(* Logix 5000 AddOnInstructionDefinition export Banner_Q90R_KD_Param_v4; software revision 33.00; part 2 of 3 *)
(* tags used below, declared in another part *)
   Q90RKD : Banner_Q90RKD_v4;
   Port_Data : Banner_IOL_Port_v4;
   Port : DINT;
   Local_Control : DINT;
   Command_Being_Processed : BOOL;
   Update_Archive : BOOL;
   Index_Write_Inprocess : DINT;
   Index_Write_Control : DINT;
   Inprocess_Index : DINT;
(* Banner_Q90R_KD_Param_v4, continued *)

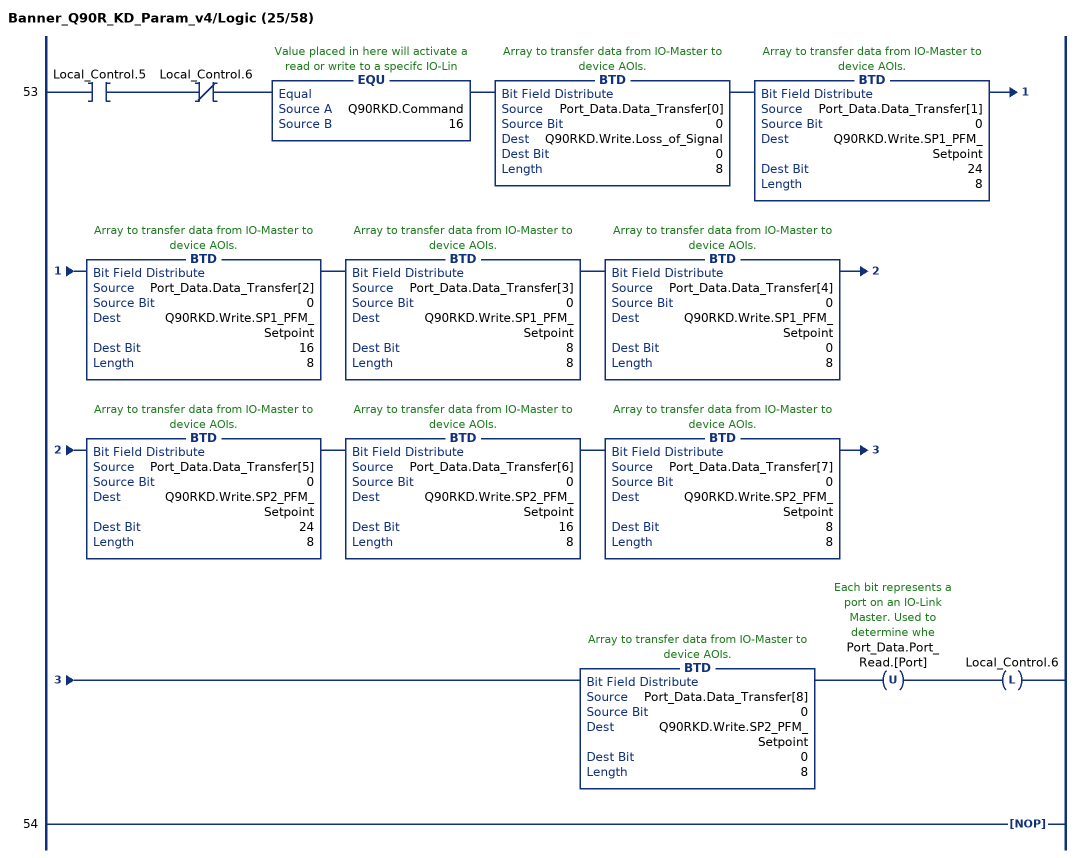
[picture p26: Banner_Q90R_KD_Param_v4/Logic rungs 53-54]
   53: XIC(Local_Control.5)XIO(Local_Control.6)EQU(Q90RKD.Command,16)BTD(Port_Data.Data_Transfer[0],0,Q90RKD.Write.Loss_of_Signal,0,8)BTD(Port_Data.Data_Transfer[1],0,Q90RKD.Write.SP1_PFM_Setpoint,24,8)BTD(Port_Data.Data_Transfer[2],0,Q90RKD.Write.SP1_PFM_Setpoint,16,8)BTD(Port_Data.Data_Transfer[3],0,Q90RKD.Write.SP1_PFM_Setpoint,8,8)BTD(Port_Data.Data_Transfer[4],0,Q90RKD.Write.SP1_PFM_Setpoint,0,8)BTD(Port_Data.Data_Transfer[5],0,Q90RKD.Write.SP2_PFM_Setpoint,24,8)BTD(Port_Data.Data_Transfer[6],0,Q90RKD.Write.SP2_PFM_Setpoint,16,8)BTD(Port_Data.Data_Transfer[7],0,Q90RKD.Write.SP2_PFM_Setpoint,8,8)BTD(Port_Data.Data_Transfer[8],0,Q90RKD.Write.SP2_PFM_Setpoint,0,8)OTU(Port_Data.Port_Read.[Port])OTL(Local_Control.6);
   54: NOP();
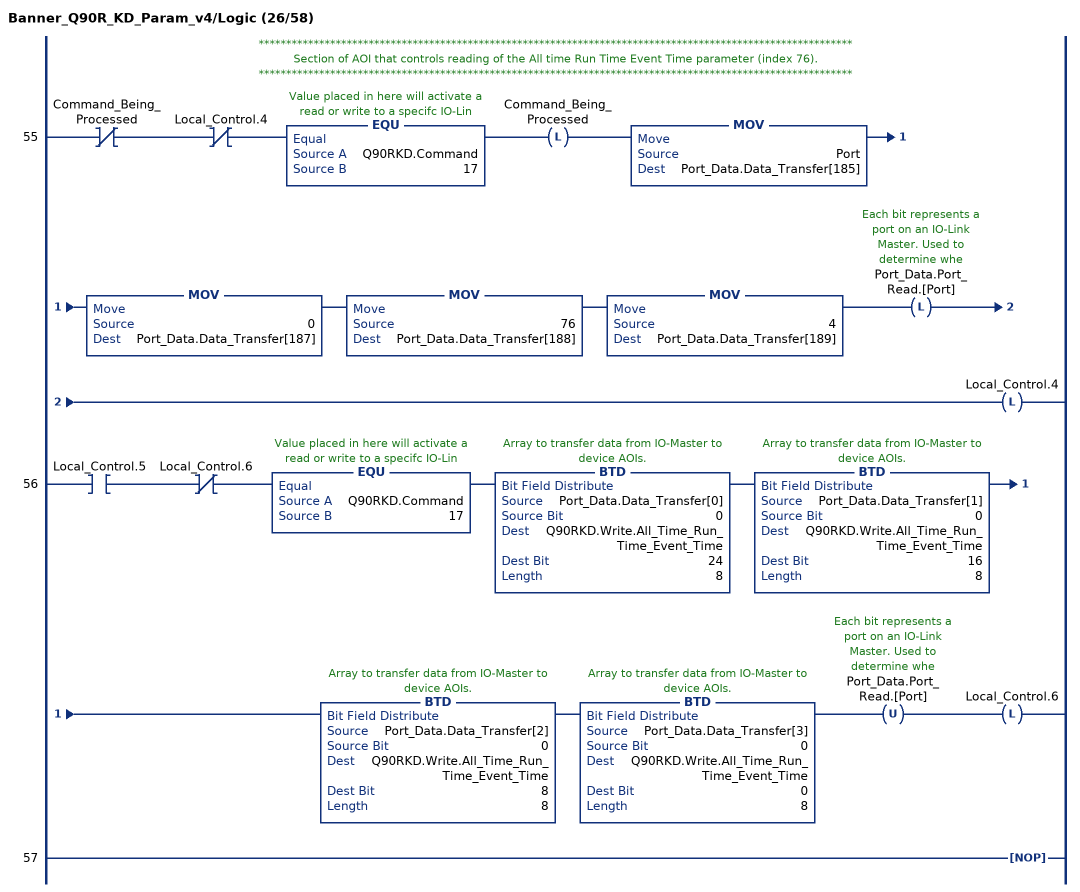
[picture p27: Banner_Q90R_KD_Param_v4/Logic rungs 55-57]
   // ************************************************************************************************************
   // Section of AOI that controls reading of the All time Run Time Event Time parameter (index 76).
   // ************************************************************************************************************
   55: XIO(Command_Being_Processed)XIO(Local_Control.4)EQU(Q90RKD.Command,17)OTL(Command_Being_Processed)MOV(Port,Port_Data.Data_Transfer[185])MOV(0,Port_Data.Data_Transfer[187])MOV(76,Port_Data.Data_Transfer[188])MOV(4,Port_Data.Data_Transfer[189])OTL(Port_Data.Port_Read.[Port])OTL(Local_Control.4);
   56: XIC(Local_Control.5)XIO(Local_Control.6)EQU(Q90RKD.Command,17)BTD(Port_Data.Data_Transfer[0],0,Q90RKD.Write.All_Time_Run_Time_Event_Time,24,8)BTD(Port_Data.Data_Transfer[1],0,Q90RKD.Write.All_Time_Run_Time_Event_Time,16,8)BTD(Port_Data.Data_Transfer[2],0,Q90RKD.Write.All_Time_Run_Time_Event_Time,8,8)BTD(Port_Data.Data_Transfer[3],0,Q90RKD.Write.All_Time_Run_Time_Event_Time,0,8)OTU(Port_Data.Port_Read.[Port])OTL(Local_Control.6);
   57: NOP();
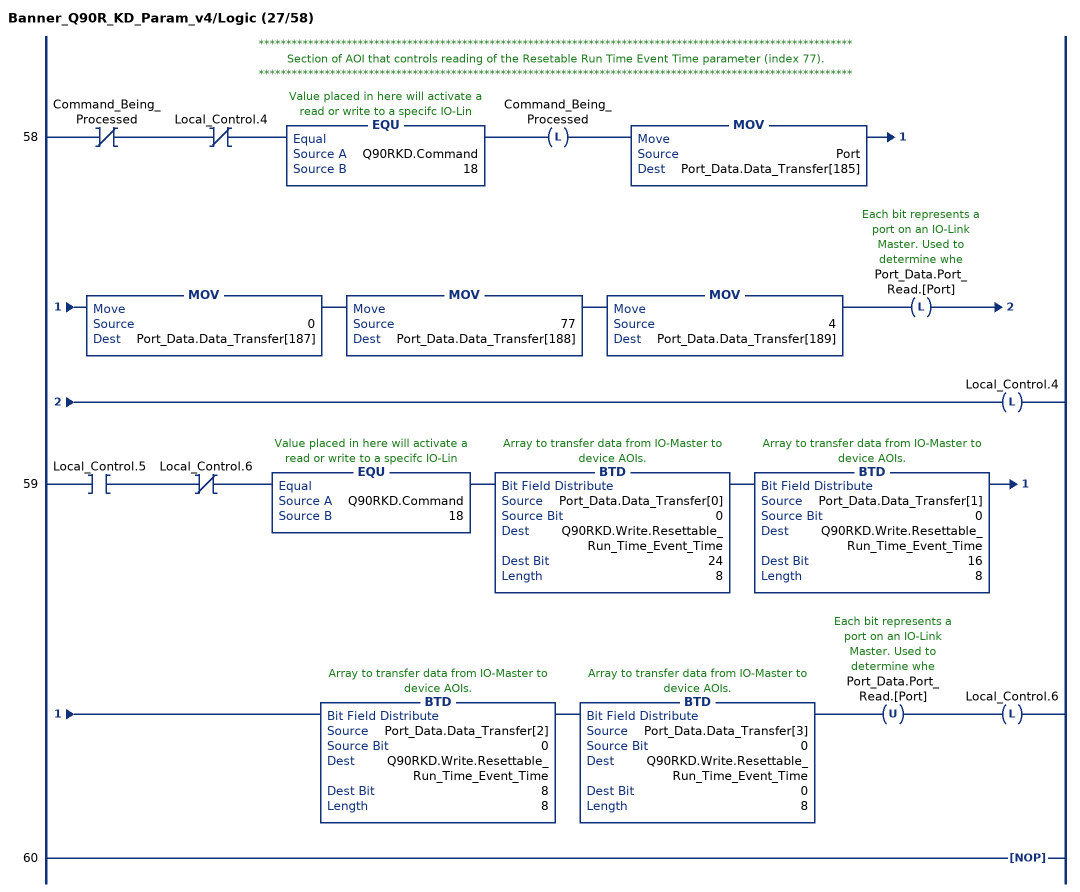
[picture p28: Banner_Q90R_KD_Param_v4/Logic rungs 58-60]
   // ************************************************************************************************************
   // Section of AOI that controls reading of the Resetable Run Time Event Time parameter (index 77).
   // ************************************************************************************************************
   58: XIO(Command_Being_Processed)XIO(Local_Control.4)EQU(Q90RKD.Command,18)OTL(Command_Being_Processed)MOV(Port,Port_Data.Data_Transfer[185])MOV(0,Port_Data.Data_Transfer[187])MOV(77,Port_Data.Data_Transfer[188])MOV(4,Port_Data.Data_Transfer[189])OTL(Port_Data.Port_Read.[Port])OTL(Local_Control.4);
   59: XIC(Local_Control.5)XIO(Local_Control.6)EQU(Q90RKD.Command,18)BTD(Port_Data.Data_Transfer[0],0,Q90RKD.Write.Resettable_Run_Time_Event_Time,24,8)BTD(Port_Data.Data_Transfer[1],0,Q90RKD.Write.Resettable_Run_Time_Event_Time,16,8)BTD(Port_Data.Data_Transfer[2],0,Q90RKD.Write.Resettable_Run_Time_Event_Time,8,8)BTD(Port_Data.Data_Transfer[3],0,Q90RKD.Write.Resettable_Run_Time_Event_Time,0,8)OTU(Port_Data.Port_Read.[Port])OTL(Local_Control.6);
   60: NOP();
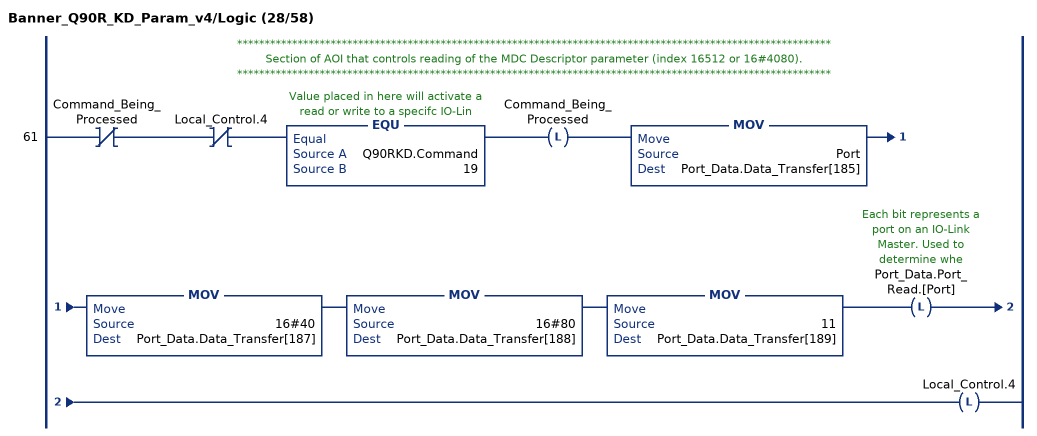
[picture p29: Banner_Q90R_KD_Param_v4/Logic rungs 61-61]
   // ************************************************************************************************************
   // Section of AOI that controls reading of the MDC Descriptor parameter (index 16512 or 16#4080).
   // ************************************************************************************************************
   61: XIO(Command_Being_Processed)XIO(Local_Control.4)EQU(Q90RKD.Command,19)OTL(Command_Being_Processed)MOV(Port,Port_Data.Data_Transfer[185])MOV(16#40,Port_Data.Data_Transfer[187])MOV(16#80,Port_Data.Data_Transfer[188])MOV(11,Port_Data.Data_Transfer[189])OTL(Port_Data.Port_Read.[Port])OTL(Local_Control.4);
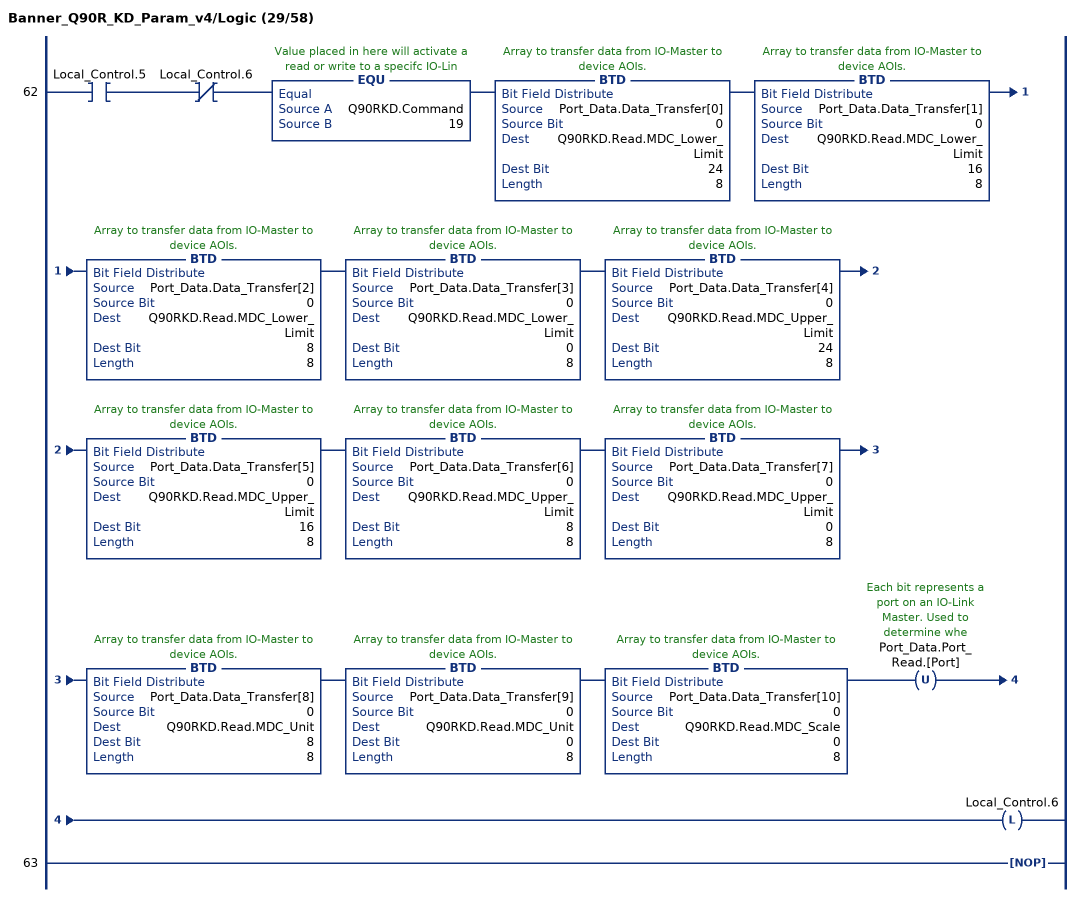
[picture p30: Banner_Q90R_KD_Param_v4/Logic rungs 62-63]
   62: XIC(Local_Control.5)XIO(Local_Control.6)EQU(Q90RKD.Command,19)BTD(Port_Data.Data_Transfer[0],0,Q90RKD.Read.MDC_Lower_Limit,24,8)BTD(Port_Data.Data_Transfer[1],0,Q90RKD.Read.MDC_Lower_Limit,16,8)BTD(Port_Data.Data_Transfer[2],0,Q90RKD.Read.MDC_Lower_Limit,8,8)BTD(Port_Data.Data_Transfer[3],0,Q90RKD.Read.MDC_Lower_Limit,0,8)BTD(Port_Data.Data_Transfer[4],0,Q90RKD.Read.MDC_Upper_Limit,24,8)BTD(Port_Data.Data_Transfer[5],0,Q90RKD.Read.MDC_Upper_Limit,16,8)BTD(Port_Data.Data_Transfer[6],0,Q90RKD.Read.MDC_Upper_Limit,8,8)BTD(Port_Data.Data_Transfer[7],0,Q90RKD.Read.MDC_Upper_Limit,0,8)BTD(Port_Data.Data_Transfer[8],0,Q90RKD.Read.MDC_Unit,8,8)BTD(Port_Data.Data_Transfer[9],0,Q90RKD.Read.MDC_Unit,0,8)BTD(Port_Data.Data_Transfer[10],0,Q90RKD.Read.MDC_Scale,0,8)OTU(Port_Data.Port_Read.[Port])OTL(Local_Control.6);
   63: NOP();
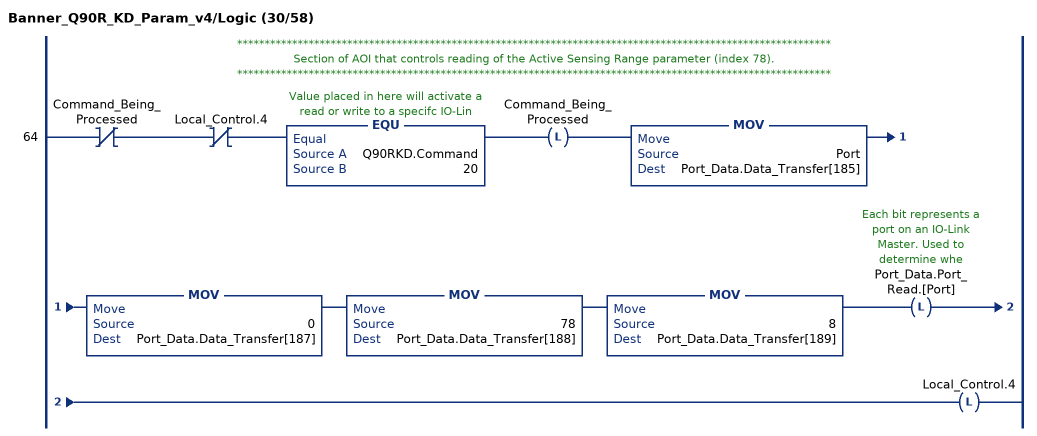
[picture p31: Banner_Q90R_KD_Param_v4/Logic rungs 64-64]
   // ************************************************************************************************************
   // Section of AOI that controls reading of the Active Sensing Range parameter (index 78).
   // ************************************************************************************************************
   64: XIO(Command_Being_Processed)XIO(Local_Control.4)EQU(Q90RKD.Command,20)OTL(Command_Being_Processed)MOV(Port,Port_Data.Data_Transfer[185])MOV(0,Port_Data.Data_Transfer[187])MOV(78,Port_Data.Data_Transfer[188])MOV(8,Port_Data.Data_Transfer[189])OTL(Port_Data.Port_Read.[Port])OTL(Local_Control.4);
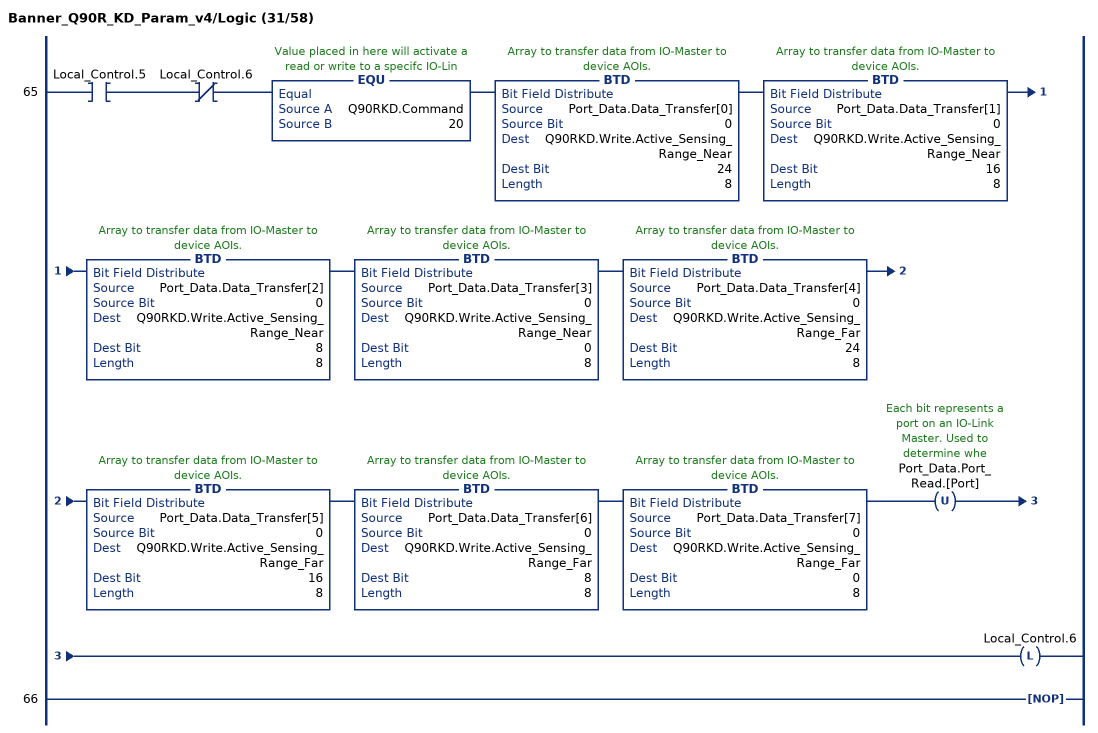
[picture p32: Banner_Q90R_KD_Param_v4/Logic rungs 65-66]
   65: XIC(Local_Control.5)XIO(Local_Control.6)EQU(Q90RKD.Command,20)BTD(Port_Data.Data_Transfer[0],0,Q90RKD.Write.Active_Sensing_Range_Near,24,8)BTD(Port_Data.Data_Transfer[1],0,Q90RKD.Write.Active_Sensing_Range_Near,16,8)BTD(Port_Data.Data_Transfer[2],0,Q90RKD.Write.Active_Sensing_Range_Near,8,8)BTD(Port_Data.Data_Transfer[3],0,Q90RKD.Write.Active_Sensing_Range_Near,0,8)BTD(Port_Data.Data_Transfer[4],0,Q90RKD.Write.Active_Sensing_Range_Far,24,8)BTD(Port_Data.Data_Transfer[5],0,Q90RKD.Write.Active_Sensing_Range_Far,16,8)BTD(Port_Data.Data_Transfer[6],0,Q90RKD.Write.Active_Sensing_Range_Far,8,8)BTD(Port_Data.Data_Transfer[7],0,Q90RKD.Write.Active_Sensing_Range_Far,0,8)OTU(Port_Data.Port_Read.[Port])OTL(Local_Control.6);
   66: NOP();
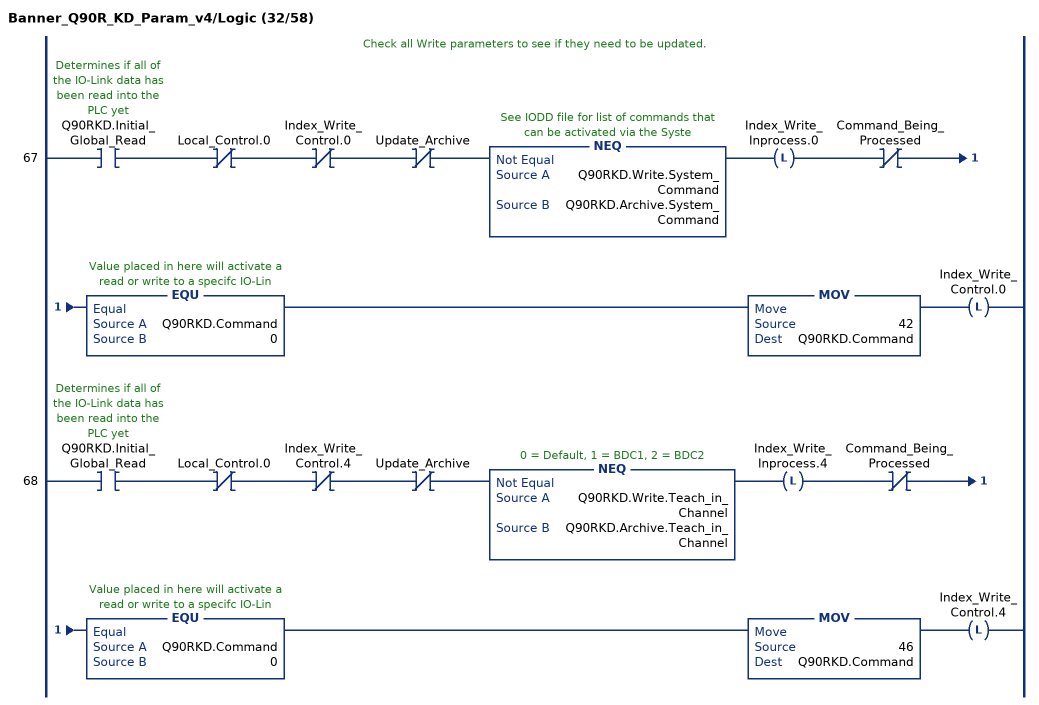
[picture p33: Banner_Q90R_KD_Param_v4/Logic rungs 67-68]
   // Check all Write parameters to see if they need to be updated.
   67: XIC(Q90RKD.Initial_Global_Read)XIO(Local_Control.0)XIO(Index_Write_Control.0)XIO(Update_Archive)NEQ(Q90RKD.Write.System_Command,Q90RKD.Archive.System_Command)OTL(Index_Write_Inprocess.0)XIO(Command_Being_Processed)EQU(Q90RKD.Command,0)MOV(42,Q90RKD.Command)OTL(Index_Write_Control.0);
   68: XIC(Q90RKD.Initial_Global_Read)XIO(Local_Control.0)XIO(Index_Write_Control.4)XIO(Update_Archive)NEQ(Q90RKD.Write.Teach_in_Channel,Q90RKD.Archive.Teach_in_Channel)OTL(Index_Write_Inprocess.4)XIO(Command_Being_Processed)EQU(Q90RKD.Command,0)MOV(46,Q90RKD.Command)OTL(Index_Write_Control.4);
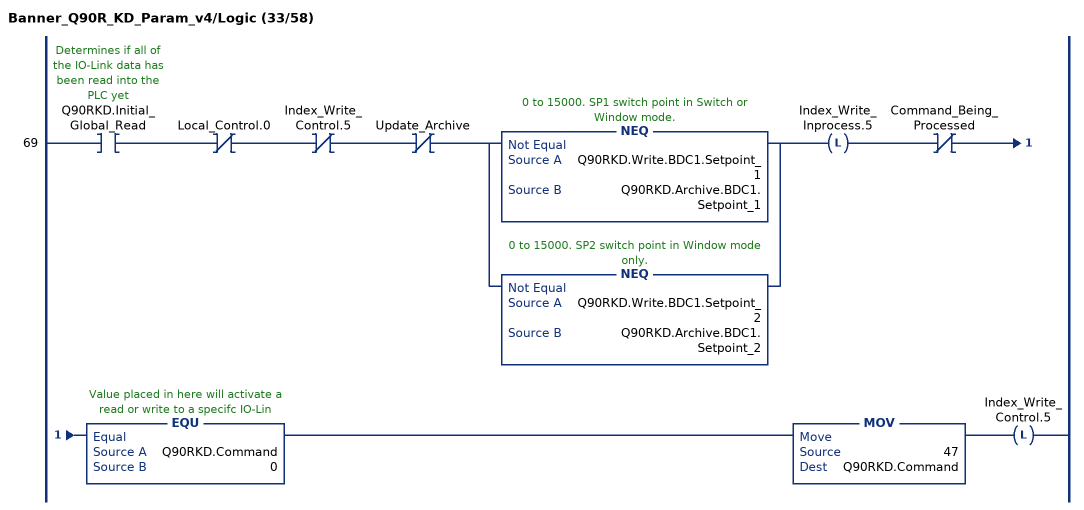
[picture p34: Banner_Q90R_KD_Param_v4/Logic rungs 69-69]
   69: XIC(Q90RKD.Initial_Global_Read)XIO(Local_Control.0)XIO(Index_Write_Control.5)XIO(Update_Archive)[NEQ(Q90RKD.Write.BDC1.Setpoint_1,Q90RKD.Archive.BDC1.Setpoint_1) ,NEQ(Q90RKD.Write.BDC1.Setpoint_2,Q90RKD.Archive.BDC1.Setpoint_2) ]OTL(Index_Write_Inprocess.5)XIO(Command_Being_Processed)EQU(Q90RKD.Command,0)MOV(47,Q90RKD.Command)OTL(Index_Write_Control.5);
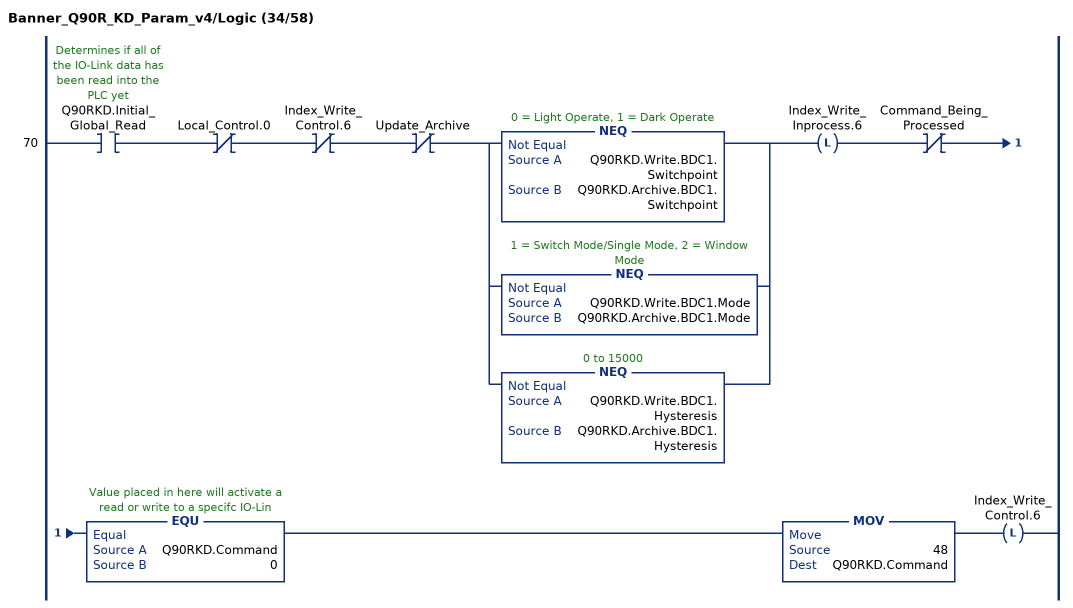
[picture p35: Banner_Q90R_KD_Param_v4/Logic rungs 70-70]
   70: XIC(Q90RKD.Initial_Global_Read)XIO(Local_Control.0)XIO(Index_Write_Control.6)XIO(Update_Archive)[NEQ(Q90RKD.Write.BDC1.Switchpoint,Q90RKD.Archive.BDC1.Switchpoint) ,NEQ(Q90RKD.Write.BDC1.Mode,Q90RKD.Archive.BDC1.Mode) ,NEQ(Q90RKD.Write.BDC1.Hysteresis,Q90RKD.Archive.BDC1.Hysteresis) ]OTL(Index_Write_Inprocess.6)XIO(Command_Being_Processed)EQU(Q90RKD.Command,0)MOV(48,Q90RKD.Command)OTL(Index_Write_Control.6);
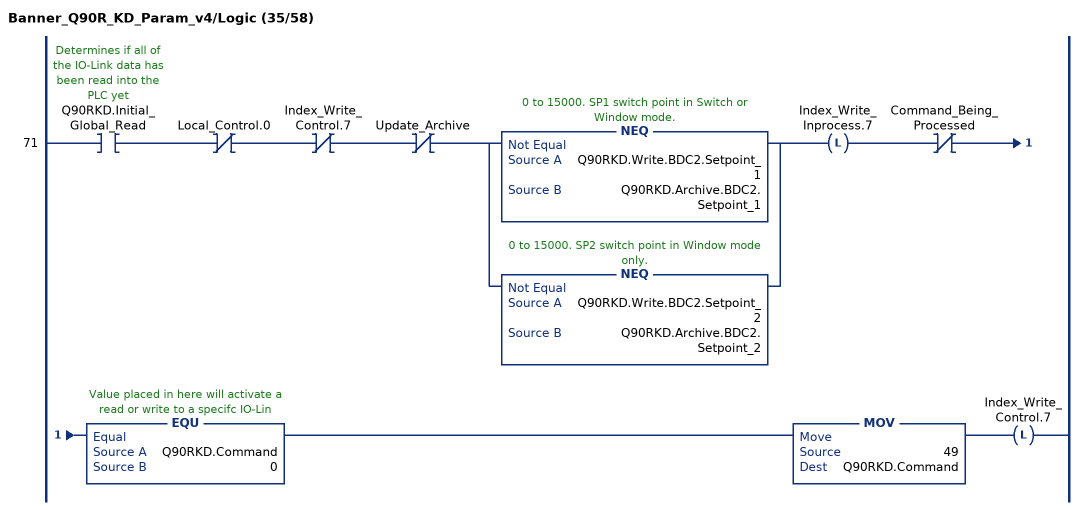
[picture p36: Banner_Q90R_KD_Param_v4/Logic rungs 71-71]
   71: XIC(Q90RKD.Initial_Global_Read)XIO(Local_Control.0)XIO(Index_Write_Control.7)XIO(Update_Archive)[NEQ(Q90RKD.Write.BDC2.Setpoint_1,Q90RKD.Archive.BDC2.Setpoint_1) ,NEQ(Q90RKD.Write.BDC2.Setpoint_2,Q90RKD.Archive.BDC2.Setpoint_2) ]OTL(Index_Write_Inprocess.7)XIO(Command_Being_Processed)EQU(Q90RKD.Command,0)MOV(49,Q90RKD.Command)OTL(Index_Write_Control.7);
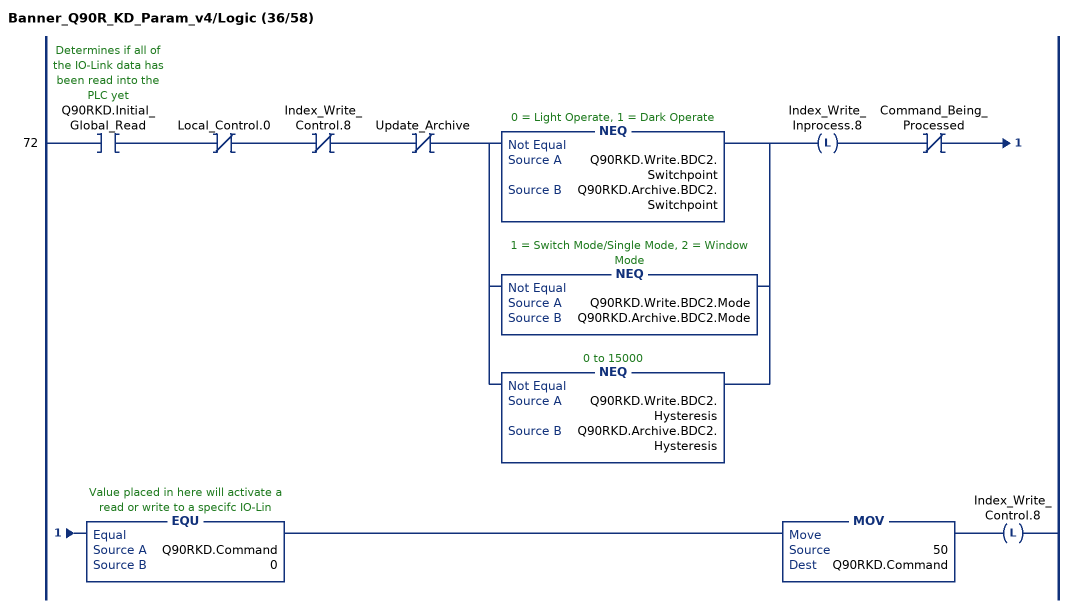
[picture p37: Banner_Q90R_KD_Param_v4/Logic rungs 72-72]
   72: XIC(Q90RKD.Initial_Global_Read)XIO(Local_Control.0)XIO(Index_Write_Control.8)XIO(Update_Archive)[NEQ(Q90RKD.Write.BDC2.Switchpoint,Q90RKD.Archive.BDC2.Switchpoint) ,NEQ(Q90RKD.Write.BDC2.Mode,Q90RKD.Archive.BDC2.Mode) ,NEQ(Q90RKD.Write.BDC2.Hysteresis,Q90RKD.Archive.BDC2.Hysteresis) ]OTL(Index_Write_Inprocess.8)XIO(Command_Being_Processed)EQU(Q90RKD.Command,0)MOV(50,Q90RKD.Command)OTL(Index_Write_Control.8);
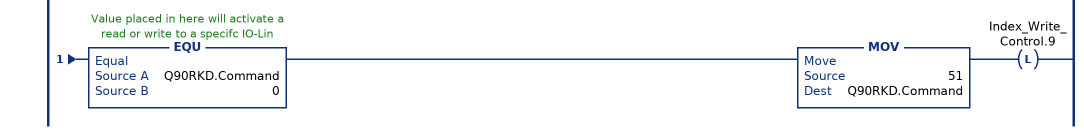
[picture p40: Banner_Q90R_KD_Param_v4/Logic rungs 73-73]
   73: XIC(Q90RKD.Initial_Global_Read)XIO(Local_Control.0)XIO(Index_Write_Control.9)XIO(Update_Archive)[NEQ(Q90RKD.Write.Config.Response_Speed,Q90RKD.Archive.Config.Response_Speed) ,NEQ(Q90RKD.Write.Config.Peak_Select_Mode,Q90RKD.Archive.Config.Peak_Select_Mode) ,NEQ(Q90RKD.Write.Config.Output_Polarity,Q90RKD.Archive.Config.Output_Polarity) ,NEQ(Q90RKD.Write.Config.Process_Data_Filter_Time,Q90RKD.Archive.Config.Process_Data_Filter_Time) ,NEQ(Q90RKD.Write.Config.Process_Data_Layout,Q90RKD.Archive.Config.Process_Data_Layout) ,NEQ(Q90RKD.Write.Config.Remote_Input_Mode,Q90RKD.Archive.Config.Remote_Input_Mode) ,NEQ(Q90RKD.Write.Config.LEDs_Disabled,Q90RKD.Archive.Config.LEDs_Disabled) ,NEQ(Q90RKD.Write.Config.Amplitude_Threshold,Q90RKD.Archive.Config.Amplitude_Threshold) ,NEQ(Q90RKD.Write.Config.Limit_Filter_Enabled,Q90RKD.Archive.Config.Limit_Filter_Enabled) ,NEQ(Q90RKD.Write.Config.Limit_Filter_Positive_Hold_Time,Q90RKD.Archive.Config.Limit_Filter_Positive_Hold_Time) ,NEQ(Q90RKD.Write.Config.Limit_Filter_Negative_Hold_Time,Q90RKD.Archive.Config.Limit_Filter_Negative_Hold_Time) ,NEQ(Q90RKD.Write.Config.Limit_Filter_Positive_Distance,Q90RKD.Archive.Config.Limit_Filter_Positive_Distance) ,NEQ(Q90RKD.Write.Config.Limit_Filter_Negative_Distance,Q90RKD.Archive.Config.Limit_Filter_Negative_Distance) ,NEQ(Q90RKD.Write.Config.Secondary_Output_Mode,Q90RKD.Archive.Config.Secondary_Output_Mode) ]OTL(Index_Write_Inprocess.9)XIO(Command_Being_Processed)EQU(Q90RKD.Command,0)MOV(51,Q90RKD.Command)OTL(Index_Write_Control.9);
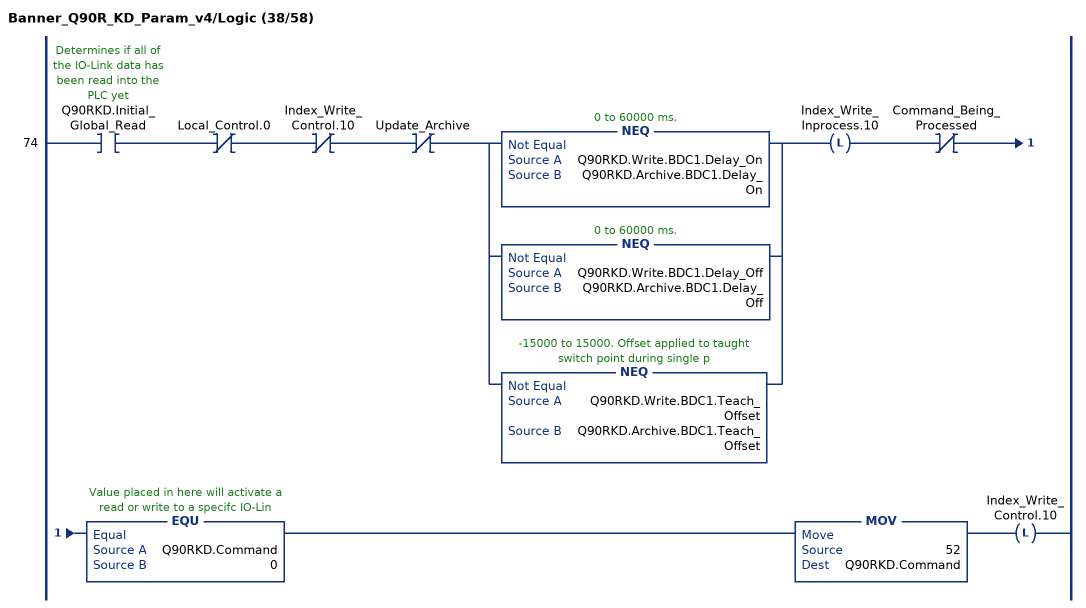
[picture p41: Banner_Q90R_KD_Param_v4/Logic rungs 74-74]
   74: XIC(Q90RKD.Initial_Global_Read)XIO(Local_Control.0)XIO(Index_Write_Control.10)XIO(Update_Archive)[NEQ(Q90RKD.Write.BDC1.Delay_On,Q90RKD.Archive.BDC1.Delay_On) ,NEQ(Q90RKD.Write.BDC1.Delay_Off,Q90RKD.Archive.BDC1.Delay_Off) ,NEQ(Q90RKD.Write.BDC1.Teach_Offset,Q90RKD.Archive.BDC1.Teach_Offset) ]OTL(Index_Write_Inprocess.10)XIO(Command_Being_Processed)EQU(Q90RKD.Command,0)MOV(52,Q90RKD.Command)OTL(Index_Write_Control.10);
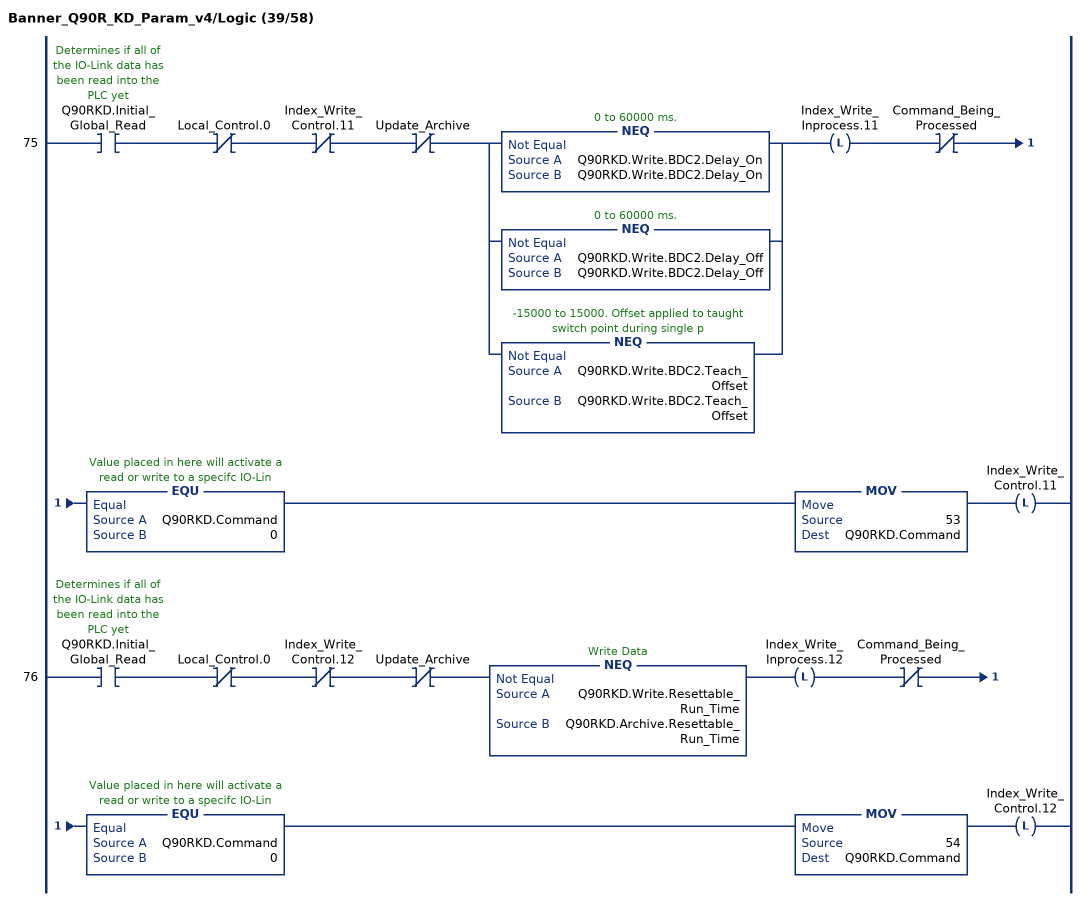
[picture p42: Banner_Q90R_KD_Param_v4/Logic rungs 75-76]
   75: XIC(Q90RKD.Initial_Global_Read)XIO(Local_Control.0)XIO(Index_Write_Control.11)XIO(Update_Archive)[NEQ(Q90RKD.Write.BDC2.Delay_On,Q90RKD.Write.BDC2.Delay_On) ,NEQ(Q90RKD.Write.BDC2.Delay_Off,Q90RKD.Write.BDC2.Delay_Off) ,NEQ(Q90RKD.Write.BDC2.Teach_Offset,Q90RKD.Write.BDC2.Teach_Offset) ]OTL(Index_Write_Inprocess.11)XIO(Command_Being_Processed)EQU(Q90RKD.Command,0)MOV(53,Q90RKD.Command)OTL(Index_Write_Control.11);
   76: XIC(Q90RKD.Initial_Global_Read)XIO(Local_Control.0)XIO(Index_Write_Control.12)XIO(Update_Archive)NEQ(Q90RKD.Write.Resettable_Run_Time,Q90RKD.Archive.Resettable_Run_Time)OTL(Index_Write_Inprocess.12)XIO(Command_Being_Processed)EQU(Q90RKD.Command,0)MOV(54,Q90RKD.Command)OTL(Index_Write_Control.12);
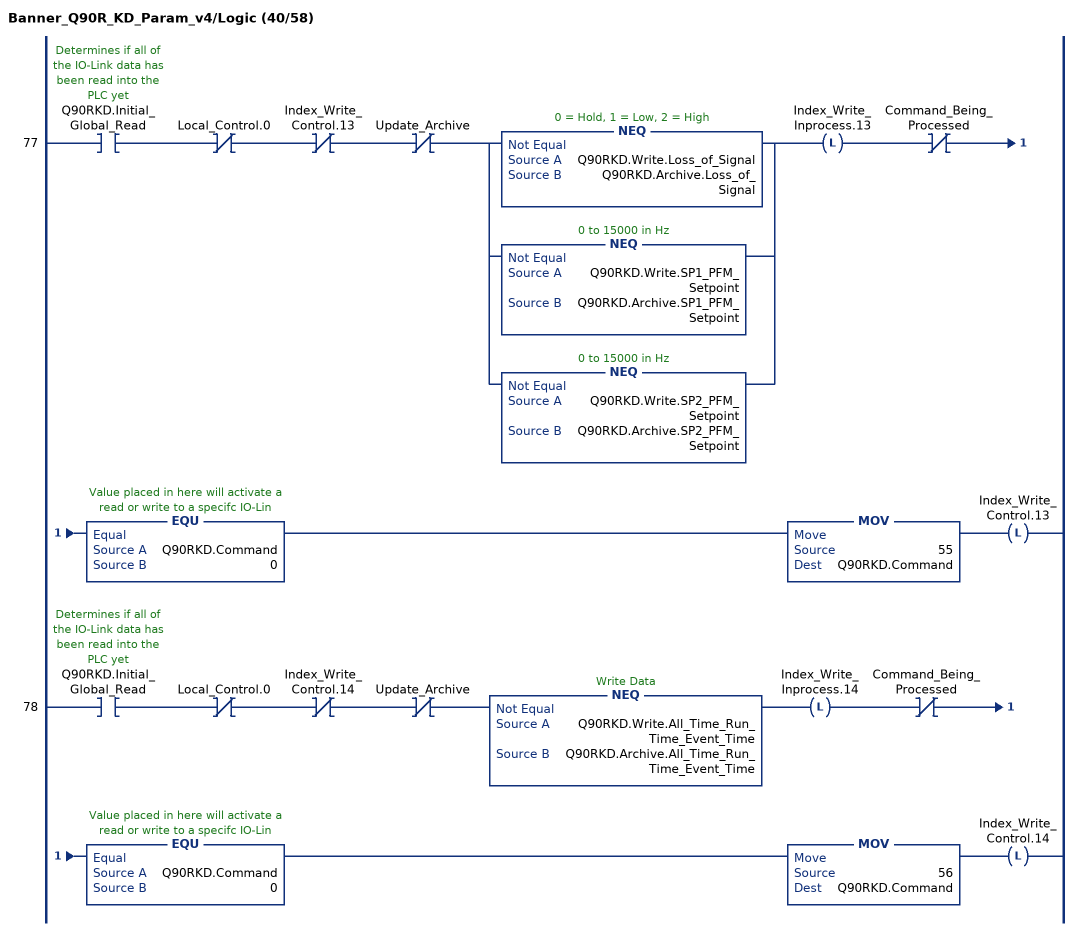
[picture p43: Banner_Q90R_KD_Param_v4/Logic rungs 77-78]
   77: XIC(Q90RKD.Initial_Global_Read)XIO(Local_Control.0)XIO(Index_Write_Control.13)XIO(Update_Archive)[NEQ(Q90RKD.Write.Loss_of_Signal,Q90RKD.Archive.Loss_of_Signal) ,NEQ(Q90RKD.Write.SP1_PFM_Setpoint,Q90RKD.Archive.SP1_PFM_Setpoint) ,NEQ(Q90RKD.Write.SP2_PFM_Setpoint,Q90RKD.Archive.SP2_PFM_Setpoint) ]OTL(Index_Write_Inprocess.13)XIO(Command_Being_Processed)EQU(Q90RKD.Command,0)MOV(55,Q90RKD.Command)OTL(Index_Write_Control.13);
   78: XIC(Q90RKD.Initial_Global_Read)XIO(Local_Control.0)XIO(Index_Write_Control.14)XIO(Update_Archive)NEQ(Q90RKD.Write.All_Time_Run_Time_Event_Time,Q90RKD.Archive.All_Time_Run_Time_Event_Time)OTL(Index_Write_Inprocess.14)XIO(Command_Being_Processed)EQU(Q90RKD.Command,0)MOV(56,Q90RKD.Command)OTL(Index_Write_Control.14);
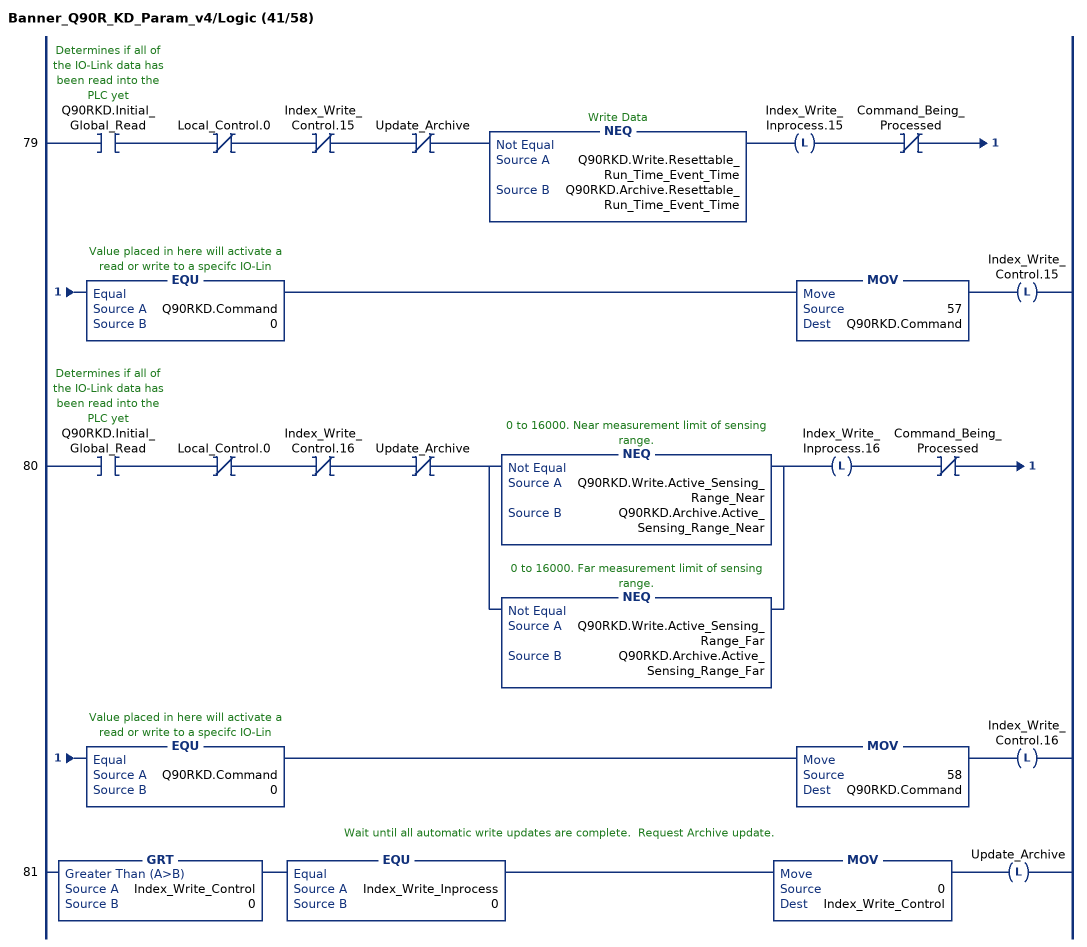
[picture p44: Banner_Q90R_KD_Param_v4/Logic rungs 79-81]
   79: XIC(Q90RKD.Initial_Global_Read)XIO(Local_Control.0)XIO(Index_Write_Control.15)XIO(Update_Archive)NEQ(Q90RKD.Write.Resettable_Run_Time_Event_Time,Q90RKD.Archive.Resettable_Run_Time_Event_Time)OTL(Index_Write_Inprocess.15)XIO(Command_Being_Processed)EQU(Q90RKD.Command,0)MOV(57,Q90RKD.Command)OTL(Index_Write_Control.15);
   80: XIC(Q90RKD.Initial_Global_Read)XIO(Local_Control.0)XIO(Index_Write_Control.16)XIO(Update_Archive)[NEQ(Q90RKD.Write.Active_Sensing_Range_Near,Q90RKD.Archive.Active_Sensing_Range_Near) ,NEQ(Q90RKD.Write.Active_Sensing_Range_Far,Q90RKD.Archive.Active_Sensing_Range_Far) ]OTL(Index_Write_Inprocess.16)XIO(Command_Being_Processed)EQU(Q90RKD.Command,0)MOV(58,Q90RKD.Command)OTL(Index_Write_Control.16);
   // Wait until all automatic write updates are complete.  Request Archive update.
   81: GRT(Index_Write_Control,0)EQU(Index_Write_Inprocess,0)MOV(0,Index_Write_Control)OTL(Update_Archive);
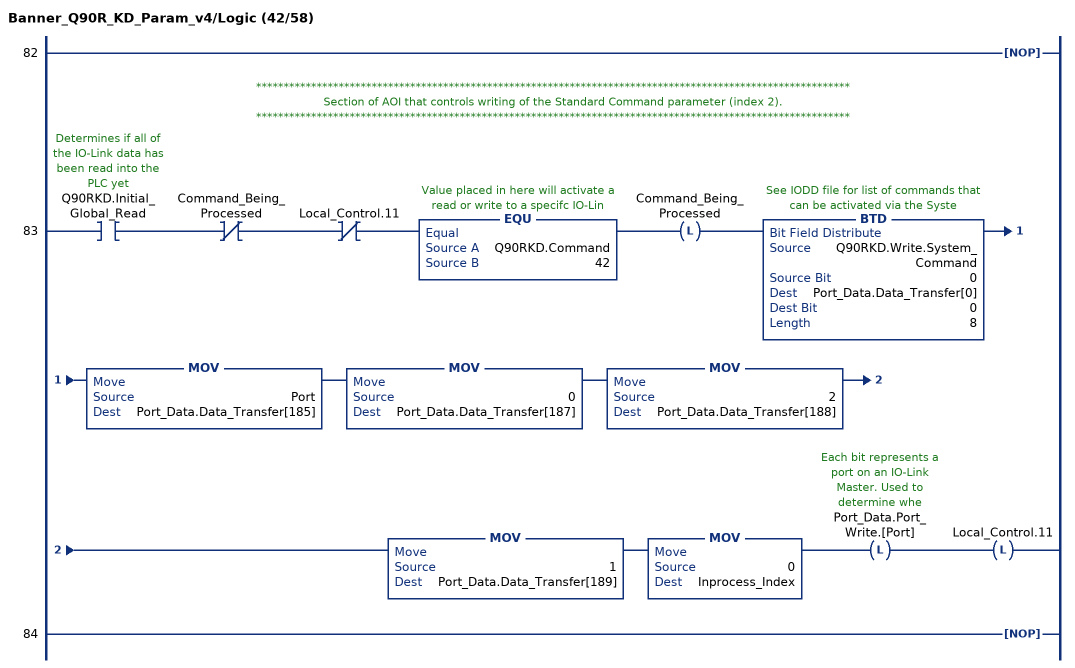
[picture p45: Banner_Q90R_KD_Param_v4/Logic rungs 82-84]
   82: NOP();
   // ************************************************************************************************************
   // Section of AOI that controls writing of the Standard Command parameter (index 2).
   // ************************************************************************************************************
   83: XIC(Q90RKD.Initial_Global_Read)XIO(Command_Being_Processed)XIO(Local_Control.11)EQU(Q90RKD.Command,42)OTL(Command_Being_Processed)BTD(Q90RKD.Write.System_Command,0,Port_Data.Data_Transfer[0],0,8)MOV(Port,Port_Data.Data_Transfer[185])MOV(0,Port_Data.Data_Transfer[187])MOV(2,Port_Data.Data_Transfer[188])MOV(1,Port_Data.Data_Transfer[189])MOV(0,Inprocess_Index)OTL(Port_Data.Port_Write.[Port])OTL(Local_Control.11);
   84: NOP();
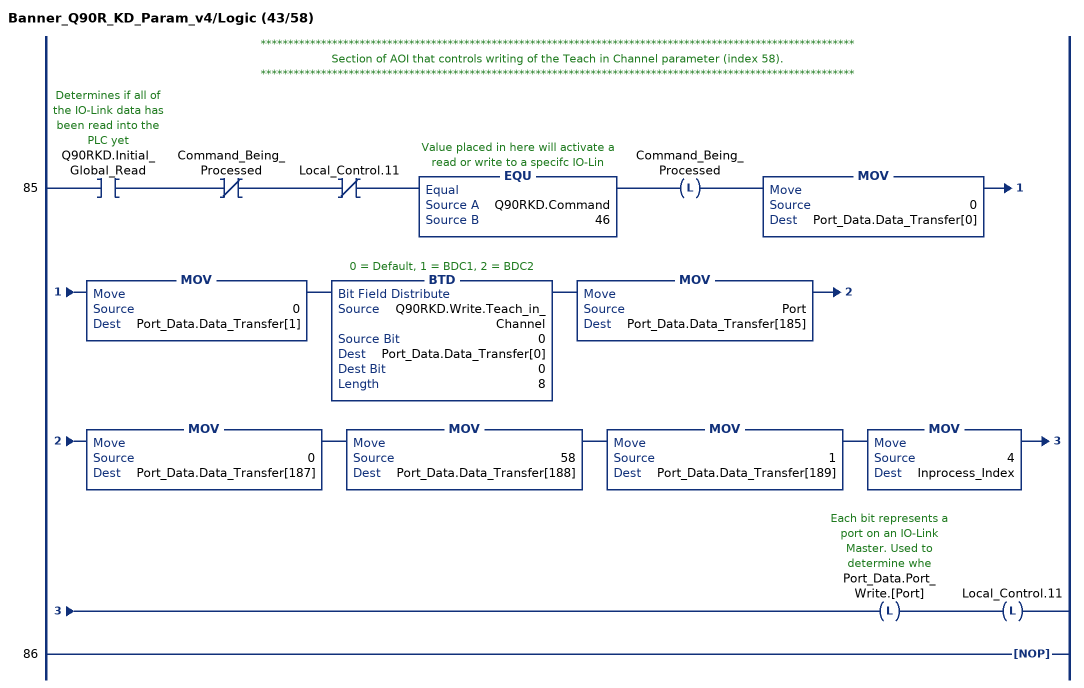
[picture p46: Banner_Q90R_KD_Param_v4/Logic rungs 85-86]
   // ************************************************************************************************************
   // Section of AOI that controls writing of the Teach in Channel parameter (index 58).
   // ************************************************************************************************************
   85: XIC(Q90RKD.Initial_Global_Read)XIO(Command_Being_Processed)XIO(Local_Control.11)EQU(Q90RKD.Command,46)OTL(Command_Being_Processed)MOV(0,Port_Data.Data_Transfer[0])MOV(0,Port_Data.Data_Transfer[1])BTD(Q90RKD.Write.Teach_in_Channel,0,Port_Data.Data_Transfer[0],0,8)MOV(Port,Port_Data.Data_Transfer[185])MOV(0,Port_Data.Data_Transfer[187])MOV(58,Port_Data.Data_Transfer[188])MOV(1,Port_Data.Data_Transfer[189])MOV(4,Inprocess_Index)OTL(Port_Data.Port_Write.[Port])OTL(Local_Control.11);
   86: NOP();
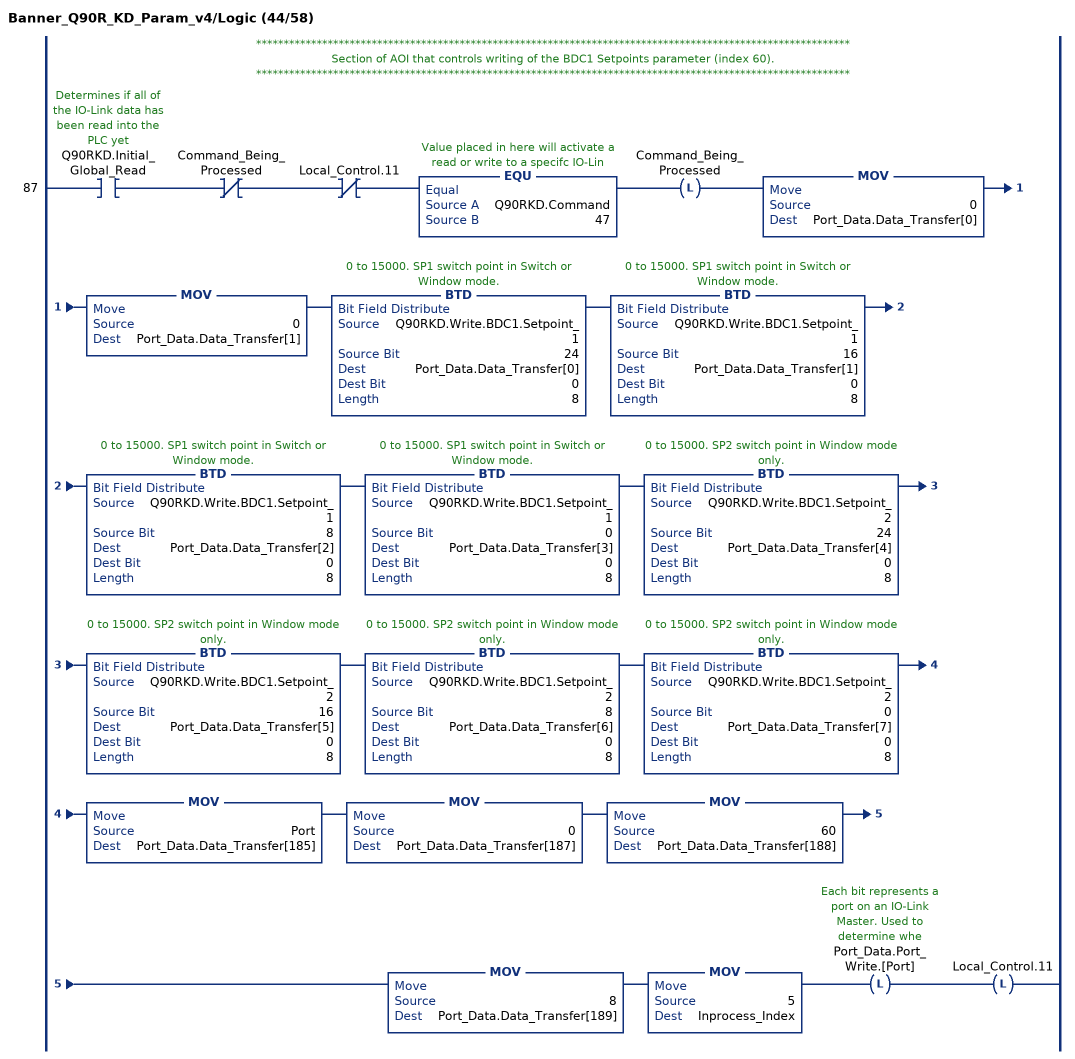
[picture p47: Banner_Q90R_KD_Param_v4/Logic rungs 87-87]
   // ************************************************************************************************************
   // Section of AOI that controls writing of the BDC1 Setpoints parameter (index 60).
   // ************************************************************************************************************
   87: XIC(Q90RKD.Initial_Global_Read)XIO(Command_Being_Processed)XIO(Local_Control.11)EQU(Q90RKD.Command,47)OTL(Command_Being_Processed)MOV(0,Port_Data.Data_Transfer[0])MOV(0,Port_Data.Data_Transfer[1])BTD(Q90RKD.Write.BDC1.Setpoint_1,24,Port_Data.Data_Transfer[0],0,8)BTD(Q90RKD.Write.BDC1.Setpoint_1,16,Port_Data.Data_Transfer[1],0,8)BTD(Q90RKD.Write.BDC1.Setpoint_1,8,Port_Data.Data_Transfer[2],0,8)BTD(Q90RKD.Write.BDC1.Setpoint_1,0,Port_Data.Data_Transfer[3],0,8)BTD(Q90RKD.Write.BDC1.Setpoint_2,24,Port_Data.Data_Transfer[4],0,8)BTD(Q90RKD.Write.BDC1.Setpoint_2,16,Port_Data.Data_Transfer[5],0,8)BTD(Q90RKD.Write.BDC1.Setpoint_2,8,Port_Data.Data_Transfer[6],0,8)BTD(Q90RKD.Write.BDC1.Setpoint_2,0,Port_Data.Data_Transfer[7],0,8)MOV(Port,Port_Data.Data_Transfer[185])MOV(0,Port_Data.Data_Transfer[187])MOV(60,Port_Data.Data_Transfer[188])MOV(8,Port_Data.Data_Transfer[189])MOV(5,Inprocess_Index)OTL(Port_Data.Port_Write.[Port])OTL(Local_Control.11);
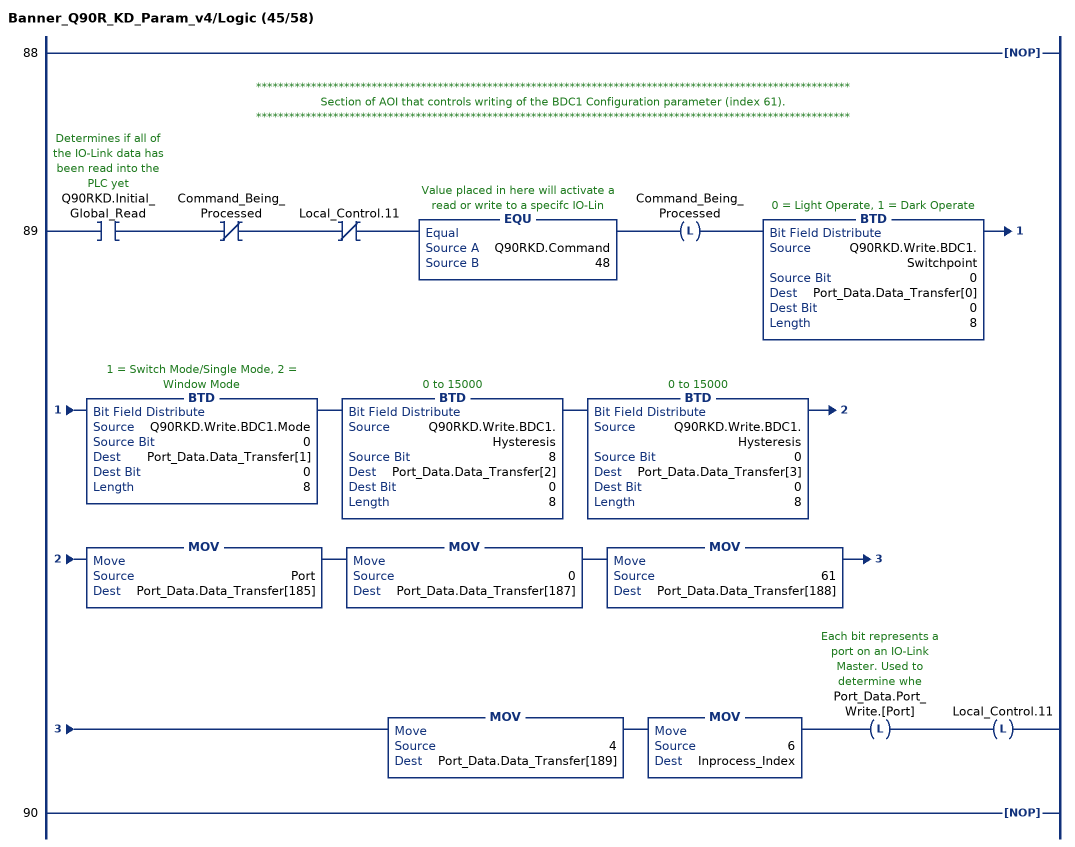
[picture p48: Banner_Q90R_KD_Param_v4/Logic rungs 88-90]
   88: NOP();
   // ************************************************************************************************************
   // Section of AOI that controls writing of the BDC1 Configuration parameter (index 61).
   // ************************************************************************************************************
   89: XIC(Q90RKD.Initial_Global_Read)XIO(Command_Being_Processed)XIO(Local_Control.11)EQU(Q90RKD.Command,48)OTL(Command_Being_Processed)BTD(Q90RKD.Write.BDC1.Switchpoint,0,Port_Data.Data_Transfer[0],0,8)BTD(Q90RKD.Write.BDC1.Mode,0,Port_Data.Data_Transfer[1],0,8)BTD(Q90RKD.Write.BDC1.Hysteresis,8,Port_Data.Data_Transfer[2],0,8)BTD(Q90RKD.Write.BDC1.Hysteresis,0,Port_Data.Data_Transfer[3],0,8)MOV(Port,Port_Data.Data_Transfer[185])MOV(0,Port_Data.Data_Transfer[187])MOV(61,Port_Data.Data_Transfer[188])MOV(4,Port_Data.Data_Transfer[189])MOV(6,Inprocess_Index)OTL(Port_Data.Port_Write.[Port])OTL(Local_Control.11);
   90: NOP();
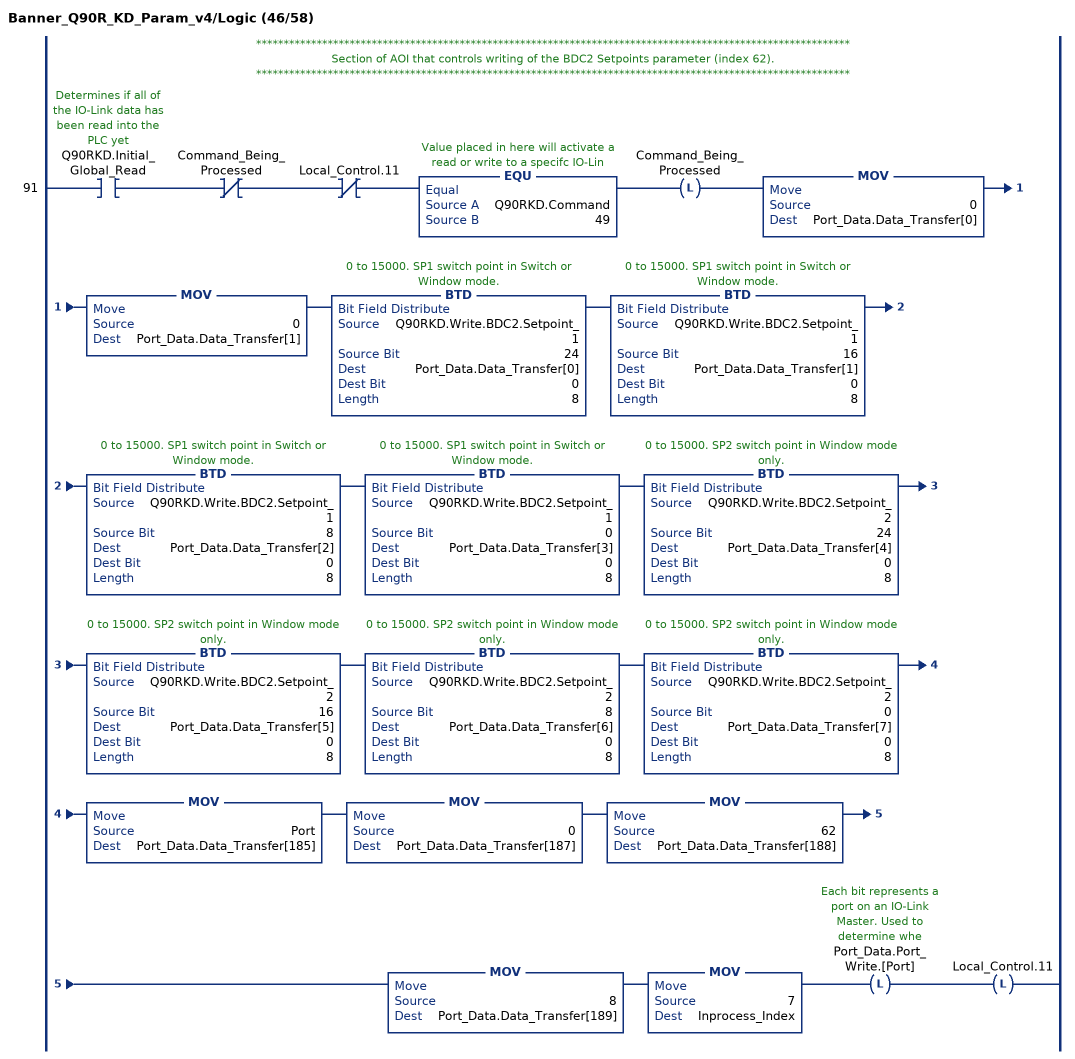
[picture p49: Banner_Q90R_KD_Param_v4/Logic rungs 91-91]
   // ************************************************************************************************************
   // Section of AOI that controls writing of the BDC2 Setpoints parameter (index 62).
   // ************************************************************************************************************
   91: XIC(Q90RKD.Initial_Global_Read)XIO(Command_Being_Processed)XIO(Local_Control.11)EQU(Q90RKD.Command,49)OTL(Command_Being_Processed)MOV(0,Port_Data.Data_Transfer[0])MOV(0,Port_Data.Data_Transfer[1])BTD(Q90RKD.Write.BDC2.Setpoint_1,24,Port_Data.Data_Transfer[0],0,8)BTD(Q90RKD.Write.BDC2.Setpoint_1,16,Port_Data.Data_Transfer[1],0,8)BTD(Q90RKD.Write.BDC2.Setpoint_1,8,Port_Data.Data_Transfer[2],0,8)BTD(Q90RKD.Write.BDC2.Setpoint_1,0,Port_Data.Data_Transfer[3],0,8)BTD(Q90RKD.Write.BDC2.Setpoint_2,24,Port_Data.Data_Transfer[4],0,8)BTD(Q90RKD.Write.BDC2.Setpoint_2,16,Port_Data.Data_Transfer[5],0,8)BTD(Q90RKD.Write.BDC2.Setpoint_2,8,Port_Data.Data_Transfer[6],0,8)BTD(Q90RKD.Write.BDC2.Setpoint_2,0,Port_Data.Data_Transfer[7],0,8)MOV(Port,Port_Data.Data_Transfer[185])MOV(0,Port_Data.Data_Transfer[187])MOV(62,Port_Data.Data_Transfer[188])MOV(8,Port_Data.Data_Transfer[189])MOV(7,Inprocess_Index)OTL(Port_Data.Port_Write.[Port])OTL(Local_Control.11);
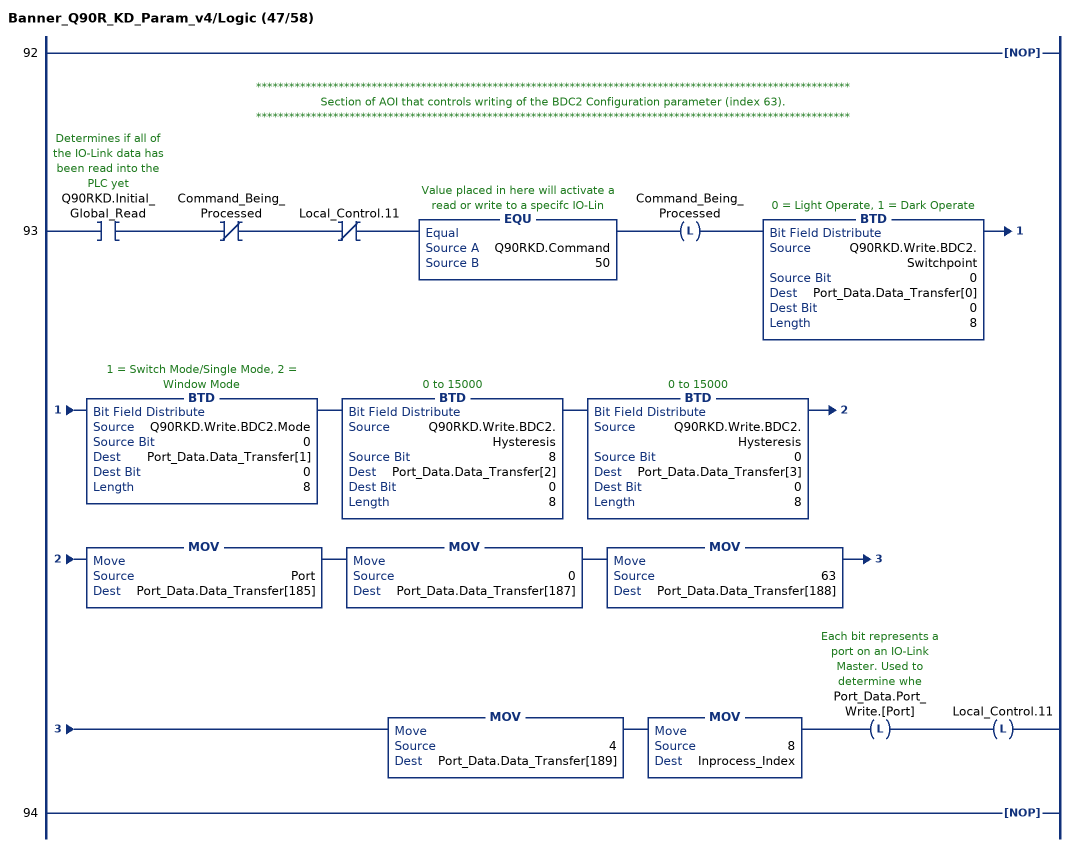
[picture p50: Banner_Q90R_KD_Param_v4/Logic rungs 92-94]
   92: NOP();
   // ************************************************************************************************************
   // Section of AOI that controls writing of the BDC2 Configuration parameter (index 63).
   // ************************************************************************************************************
   93: XIC(Q90RKD.Initial_Global_Read)XIO(Command_Being_Processed)XIO(Local_Control.11)EQU(Q90RKD.Command,50)OTL(Command_Being_Processed)BTD(Q90RKD.Write.BDC2.Switchpoint,0,Port_Data.Data_Transfer[0],0,8)BTD(Q90RKD.Write.BDC2.Mode,0,Port_Data.Data_Transfer[1],0,8)BTD(Q90RKD.Write.BDC2.Hysteresis,8,Port_Data.Data_Transfer[2],0,8)BTD(Q90RKD.Write.BDC2.Hysteresis,0,Port_Data.Data_Transfer[3],0,8)MOV(Port,Port_Data.Data_Transfer[185])MOV(0,Port_Data.Data_Transfer[187])MOV(63,Port_Data.Data_Transfer[188])MOV(4,Port_Data.Data_Transfer[189])MOV(8,Inprocess_Index)OTL(Port_Data.Port_Write.[Port])OTL(Local_Control.11);
   94: NOP();
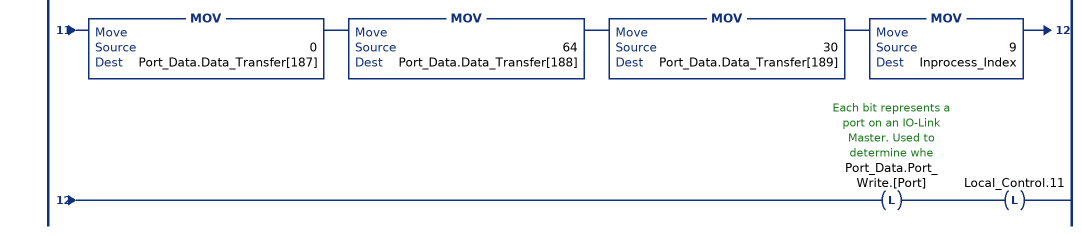
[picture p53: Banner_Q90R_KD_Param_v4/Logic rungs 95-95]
   // ************************************************************************************************************
   // Section of AOI that controls writing of the Configuration parameter (index 64).
   // ************************************************************************************************************
   95: XIC(Q90RKD.Initial_Global_Read)XIO(Command_Being_Processed)XIO(Local_Control.11)EQU(Q90RKD.Command,51)OTL(Command_Being_Processed)BTD(Q90RKD.Write.Config.Response_Speed,0,Port_Data.Data_Transfer[0],0,8)BTD(Q90RKD.Write.Config.Peak_Select_Mode,0,Port_Data.Data_Transfer[1],0,8)BTD(Q90RKD.Write.Config.Output_Polarity,0,Port_Data.Data_Transfer[2],0,8)BTD(Q90RKD.Write.Config.Process_Data_Filter_Time,8,Port_Data.Data_Transfer[3],0,8)BTD(Q90RKD.Write.Config.Process_Data_Filter_Time,0,Port_Data.Data_Transfer[4],0,8)BTD(Q90RKD.Write.Config.Process_Data_Layout,0,Port_Data.Data_Transfer[5],0,8)BTD(Q90RKD.Write.Config.Remote_Input_Mode,0,Port_Data.Data_Transfer[6],0,8)BTD(Q90RKD.Write.Config.LEDs_Disabled,0,Port_Data.Data_Transfer[7],0,8)BTD(Q90RKD.Write.Config.Amplitude_Threshold,24,Port_Data.Data_Transfer[8],0,8)BTD(Q90RKD.Write.Config.Amplitude_Threshold,16,Port_Data.Data_Transfer[9],0,8)BTD(Q90RKD.Write.Config.Amplitude_Threshold,8,Port_Data.Data_Transfer[10],0,8)BTD(Q90RKD.Write.Config.Amplitude_Threshold,0,Port_Data.Data_Transfer[11],0,8)BTD(Q90RKD.Write.Config.Limit_Filter_Enabled,0,Port_Data.Data_Transfer[12],0,8)BTD(Q90RKD.Write.Config.Limit_Filter_Positive_Hold_Time,24,Port_Data.Data_Transfer[13],0,8)BTD(Q90RKD.Write.Config.Limit_Filter_Positive_Hold_Time,16,Port_Data.Data_Transfer[14],0,8)BTD(Q90RKD.Write.Config.Limit_Filter_Positive_Hold_Time,8,Port_Data.Data_Transfer[15],0,8)BTD(Q90RKD.Write.Config.Limit_Filter_Positive_Hold_Time,0,Port_Data.Data_Transfer[16],0,8)BTD(Q90RKD.Write.Config.Limit_Filter_Negative_Hold_Time,24,Port_Data.Data_Transfer[17],0,8)BTD(Q90RKD.Write.Config.Limit_Filter_Negative_Hold_Time,16,Port_Data.Data_Transfer[18],0,8)BTD(Q90RKD.Write.Config.Limit_Filter_Negative_Hold_Time,8,Port_Data.Data_Transfer[19],0,8)BTD(Q90RKD.Write.Config.Limit_Filter_Negative_Hold_Time,0,Port_Data.Data_Transfer[20],0,8)BTD(Q90RKD.Write.Config.Limit_Filter_Positive_Distance,24,Port_Data.Data_Transfer[21],0,8)BTD(Q90RKD.Write.Config.Limit_Filter_Positive_Distance,16,Port_Data.Data_Transfer[22],0,8)BTD(Q90RKD.Write.Config.Limit_Filter_Positive_Distance,8,Port_Data.Data_Transfer[23],0,8)BTD(Q90RKD.Write.Config.Limit_Filter_Positive_Distance,0,Port_Data.Data_Transfer[24],0,8)BTD(Q90RKD.Write.Config.Limit_Filter_Negative_Distance,24,Port_Data.Data_Transfer[25],0,8)BTD(Q90RKD.Write.Config.Limit_Filter_Negative_Distance,16,Port_Data.Data_Transfer[26],0,8)BTD(Q90RKD.Write.Config.Limit_Filter_Negative_Distance,8,Port_Data.Data_Transfer[27],0,8)BTD(Q90RKD.Write.Config.Limit_Filter_Negative_Distance,0,Port_Data.Data_Transfer[28],0,8)BTD(Q90RKD.Write.Config.Secondary_Output_Mode,0,Port_Data.Data_Transfer[29],0,8)MOV(Port,Port_Data.Data_Transfer[185])MOV(0,Port_Data.Data_Transfer[187])MOV(64,Port_Data.Data_Transfer[188])MOV(30,Port_Data.Data_Transfer[189])MOV(9,Inprocess_Index)OTL(Port_Data.Port_Write.[Port])OTL(Local_Control.11);
